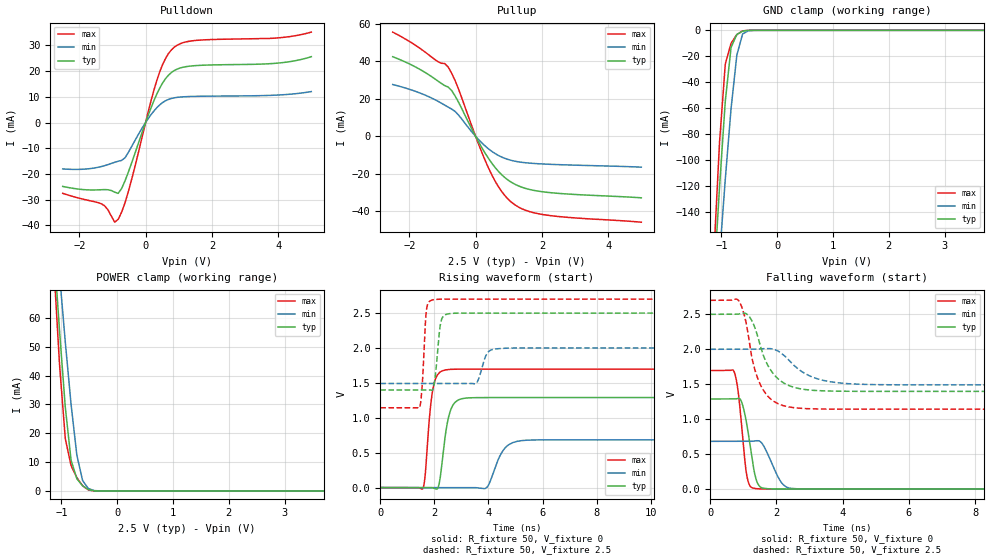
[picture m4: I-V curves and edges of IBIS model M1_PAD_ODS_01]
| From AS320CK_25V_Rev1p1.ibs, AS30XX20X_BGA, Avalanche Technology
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[Model] M1_PAD_ODS_01
Model_type I/O
Enable   Active-High
Vinl  =  0.7
Vinh  =  1.8
Vmeas =  1.25
Cref  =  30e-12
| Capacitance  typ   min   max
C_comp   1.568193e-12   1.472592e-12   1.715469e-12
| Variables   typ   min   max
[GND Clamp Reference]   0   0   0
[POWER Clamp Reference]   2.5   2   2.7
[Pulldown Reference]   0   0   0
[Pullup Reference]   2.5   2   2.7
[Temperature Range]   25   125   -40
[Voltage Range]   2.5   2   2.7
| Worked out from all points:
|   slope of the pulldown table from 0 to 0.375 V, typ, clamps not added: 31.1 ohm
|   slope of the pullup table from 0 to 0.375 V, typ, clamps not added: 33 ohm
|   GND clamp passes 1 mA (typ) near -0.64 V on its own axis
|   POWER clamp passes 1 mA (typ) near -0.56 V on its own axis
|   falling waveform, R_fixture 50, V_fixture 0: 20-80 % time 264ps typ, 400ps min, 208ps max; typ from 1.29 V to 0 V
|   falling waveform, R_fixture 50, V_fixture 2.5: 20-80 % time 592ps typ, 885ps min, 478ps max; typ from 2.5 V to 1.4 V
|   rising waveform, R_fixture 50, V_fixture 0: 20-80 % time 286ps typ, 462ps min, 228ps max; typ from 0 V to 1.29 V
|   rising waveform, R_fixture 50, V_fixture 2.5: 20-80 % time 162ps typ, 248ps min, 124ps max; typ from 1.4 V to 2.5 V
[GND Clamp]
| Voltage   I(typ)   I(min)   I(max)
-2.5V     -1.297A    -1.146A    -1.538A
-1.138V   -195.9mA   -238.3mA   -175.2mA
-1.034V   -121.2mA   -175.1mA   -86.57mA
-931mV    -54.79mA   -114.9mA   -26.01mA
-827.6mV  -13.15mA   -60.41mA   -9.967mA
-724.1mV  -3.205mA   -19.15mA   -3.28mA
-620.7mV  -615.3uA   -2.798mA   -407.6uA
-517.2mV  -34.39uA   -319.4uA   -6.513uA
-413.8mV  -821.3nA   -24.43uA   -50.96nA
5V        0A         0A         0A
[POWER Clamp]
| Voltage   I(typ)   I(min)   I(max)
-2.5V     511mA      454.9mA    606.6mA
-1.138V   84.76mA    99.9mA     78.64mA
-1.034V   55.67mA    75.27mA    43.94mA
-931mV    29.07mA    51.7mA     18.16mA
-827.6mV  10.68mA    30.08mA    8.788mA
-724.1mV  4.238mA    12.45mA    4.618mA
-620.7mV  1.771mA    3.587mA    1.776mA
-517.2mV  465uA      837.9uA    329.7uA
-413.8mV  47.65uA    120.2uA    11.19uA
-310.3mV  1.515uA    11.72uA    116.8nA
5V        0A         0A         0A
[Pulldown]
| Voltage   I(typ)   I(min)   I(max)
-2.5V     -24.87mA   -18.07mA   -27.57mA
-1.345V   -26.16mA   -17.16mA   -31.56mA
-1.138V   -26.16mA   -16.39mA   -33.92mA
-931mV    -27.1mA    -15.47mA   -38.79mA
-827.6mV  -27.57mA   -15.06mA   -37.67mA
-517.2mV  -19.21mA   -11.59mA   -26.74mA
344.8mV   11.25mA    5.851mA    16.61mA
603.4mV   17.11mA    8.493mA    24.99mA
948.3mV   20.78mA    9.791mA    30.07mA
1.638V    22.25mA    10.22mA    32.08mA
3.99V     23.14mA    10.7mA     32.95mA
5V        25.64mA    12.06mA    35.21mA
[Pullup]
| Voltage   I(typ)   I(min)   I(max)
-2.5V     42.46mA    27.63mA    55.6mA
-1.552V   34.39mA    22.21mA    45.33mA
-827.6mV  26.27mA    15.57mA    37mA
-724.1mV  24.47mA    14.55mA    33.72mA
-517.2mV  18.31mA    11.42mA    25.35mA
86.21mV   -2.828mA   -1.659mA   -4.01mA
431mV     -12.86mA   -7.26mA    -18.44mA
775.9mV   -20.29mA   -10.98mA   -29.17mA
1.121V    -24.94mA   -13.02mA   -35.71mA
1.552V    -28.01mA   -14.18mA   -39.73mA
2.069V    -29.69mA   -14.79mA   -41.84mA
5V        -32.81mA   -16.45mA   -45.81mA
[Ramp]
dV/dt_r   0.773451/0.285827n  0.410287/0.461553n  1.01797/0.227987n
dV/dt_f   0.661206/0.592287n  0.305568/0.885073n  0.934101/0.477866n
R_load = 50
[Falling Waveform]
R_fixture = 50
V_fixture = 0
V_fixture_min = 0
V_fixture_max = 0
| Time   V(typ)   V(min)   V(max)
0s        1.289V     683.8mV    1.697V
722.1ps   1.29V      684.2mV    1.678V
850.3ps   1.298V     684.2mV    1.364V
973.2ps   1.209V     684.3mV    770.5mV
1.106ns   916.6mV    684.3mV    184.4mV
1.341ns   222mV      688.2mV    10.45mV
1.551ns   20.93mV    662mV      2.925mV
2.147ns   1.244mV    95.58mV    475.4uV
2.573ns   621uV      6.282mV    465.1uV
21.88ns   -9.112nV   105.1nV    -45.88nV
[Falling Waveform]
R_fixture = 50
V_fixture = 2.5
V_fixture_min = 2
V_fixture_max = 2.7
| Time   V(typ)   V(min)   V(max)
0s        2.5V       2V         2.7V
868.6ps   2.505V     2V         2.688V
1.048ns   2.515V     2V         2.451V
1.188ns   2.462V     2V         2.075V
1.493ns   2.083V     2.005V     1.514V
1.852ns   1.683V     2.007V     1.279V
2.373ns   1.482V     1.844V     1.175V
3.235ns   1.409V     1.578V     1.147V
4.523ns   1.399V     1.5V       1.144V
21.88ns   1.398V     1.491V     1.143V
[Rising Waveform]
R_fixture = 50
V_fixture = 0
V_fixture_min = 0
V_fixture_max = 0
| Time   V(typ)   V(min)   V(max)
0s        2.717nV    63.35nV    2.393nV
1.572ns   -650.4uV   -323.5uV   -16.16mV
1.958ns   -6.907mV   -402.9uV   1.436V
2.181ns   60.06mV    -448.8uV   1.644V
2.419ns   784.3mV    -497.9uV   1.686V
2.875ns   1.252V     -591.7uV   1.696V
3.898ns   1.289V     -10.27mV   1.696V
4.565ns   1.289V     543.2mV    1.696V
5.218ns   1.289V     671.9mV    1.696V
21.88ns   1.289V     683.8mV    1.697V
[Rising Waveform]
R_fixture = 50
V_fixture = 2.5
V_fixture_min = 2
V_fixture_max = 2.7
| Time   V(typ)   V(min)   V(max)
0s        1.398V     1.491V     1.143V
1.455ns   1.399V     1.491V     1.15V
1.545ns   1.399V     1.491V     1.432V
1.71ns    1.399V     1.491V     2.55V
1.972ns   1.441V     1.491V     2.691V
2.236ns   2.362V     1.491V     2.699V
2.57ns    2.492V     1.491V     2.699V
3.539ns   2.499V     1.49V      2.699V
4.437ns   2.499V     1.992V     2.699V
21.88ns   2.5V       2V         2.7V
